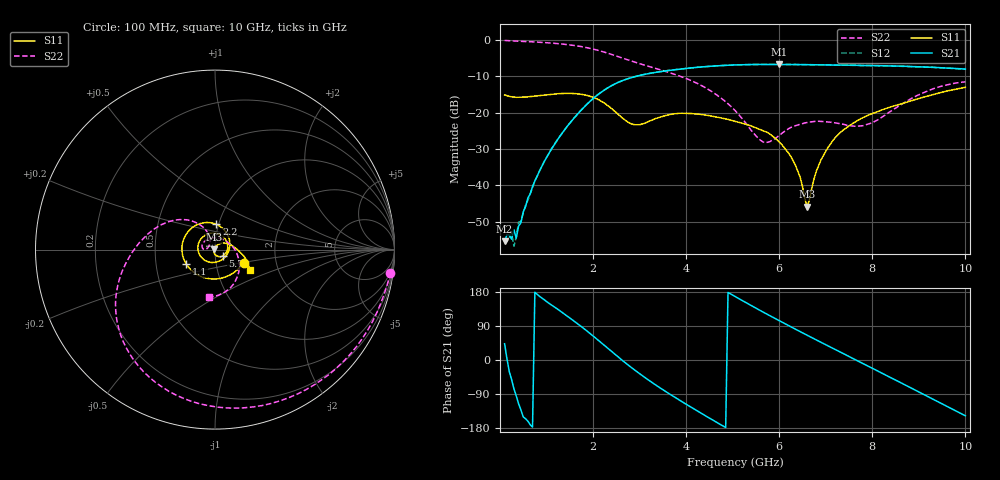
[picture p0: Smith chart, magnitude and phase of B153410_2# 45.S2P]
!  2-Port S-parameters saved by WinCal
! VAR MeasName=S-Parameters (CALIBRATED_DATA) read from VNA (N5245A)
! VAR MeasDate=2016-12-23 10:01:41
! VAR NAME=B153410_2# 45
! VAR FILENAME=B153410_2# 45.S2P
! VAR DATE=2016-12-23 10:01:41
! VAR PHYS_PORTS=1,2
# Hz S DB R 50
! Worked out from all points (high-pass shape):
!   199 points, 100 MHz to 10 GHz, reference 50 ohm
!   highest |S21| = -6.71 dB at 6 GHz (marker M1); lowest = -55.4 dB at 100 MHz (marker M2)
!   |S21| within 3 dB of the highest: 3.015 GHz to end of sweep
!   lowest |S11| = -45.9 dB at 6.6 GHz (marker M3), VSWR 1.01, Z = 49.5 + j0.0838 ohm
!   |S11| at or under -10 dB: start of sweep to end of sweep
!   |S22| runs from -28.2 to -0.1 dB; largest |S21 - S12| = 0.0036
!   S11 on the Smith chart (normalised r, x): 100 MHz: 1.36, -0.20; 1.1 GHz: 0.72, -0.12; 2.2 GHz: 0.97, +0.28; 5.7 GHz: 1.08, -0.08; 10 GHz: 1.43, -0.34
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1e8  -15.11 -24.2  -55.36 42.9  -54.74 39.6  -0.13 -7.5
2.5e8  -15.63 -51.2  -54.77 -51.4  -53.15 -42.5  -0.25 -17.6
3e8  -15.68 -59.5  -52.16 -75.8  -56.69 -79.6  -0.28 -21.0
3.5e8  -15.76 -67.0  -54.48 -94.7  -54.17 -86.6  -0.31 -24.3
6e8  -15.64 -100.7  -43.43 -161.3  -44.07 -160.9  -0.45 -40.8
1.1e9  -14.94 -152.7  -30.14 145.7  -30.05 145.8  -0.84 -73.2
1.75e9  -14.93 143.2  -19.21 88.0  -19.21 88.1  -1.82 -114.2
2.2e9  -17.00 87.0  -14.12 43.0  -14.13 43.2  -3.19 -140.8
2.85e9  -23.17 -37.3  -10.26 -22.3  -10.23 -22.1  -5.89 -170.5
3.4e9  -21.40 -143.6  -8.80 -70.3  -8.78 -70.2  -8.03 169.7
4.15e9  -20.27 125.7  -7.62 -127.9  -7.62 -127.9  -11.40 141.9
5.05e9  -22.36 25.6  -6.86 167.6  -6.86 167.8  -19.38 114.2
5.7e9  -25.15 -40.6  -6.73 123.4  -6.73 123.5  -28.25 150.9
6e9  -28.07 -69.5  -6.71 104.0  -6.70 104.0  -26.24 176.2
6.35e9  -34.46 -106.0  -6.76 81.2  -6.75 81.4  -23.56 176.6
6.6e9  -45.86 170.4  -6.77 65.5  -6.78 65.5  -22.69 168.4
6.7e9  -40.79 106.8  -6.79 59.1  -6.80 59.1  -22.50 164.3
6.9e9  -32.89 73.6  -6.82 46.5  -6.84 46.6  -22.39 154.3
7.2e9  -26.91 48.8  -6.89 27.8  -6.89 27.9  -22.78 134.9
8.35e9  -18.61 3.1  -7.14 -43.7  -7.14 -43.5  -19.96 8.6
9.15e9  -15.56 -13.3  -7.42 -93.7  -7.45 -93.7  -14.21 -50.2
1e10  -13.00 -30.6  -8.00 -147.2  -8.03 -146.8  -11.52 -97.4
